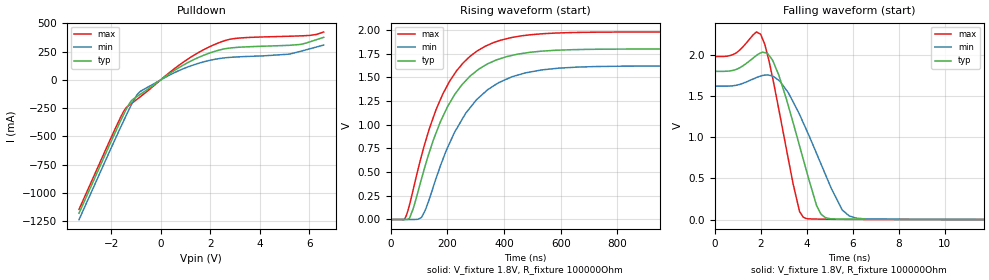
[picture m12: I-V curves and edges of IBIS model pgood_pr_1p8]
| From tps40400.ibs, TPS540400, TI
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|   pgood_pr_1p8 Model
[Model]   pgood_pr_1p8
Model_type   Open_drain
Polarity   Non-Inverting
Vmeas = 0.9
Vref = 1.8
Cref = 1pF
Rref = 100000
|   typ   min   max
C_comp   1.431pF   1.292pF   1.756pF
[Voltage Range]   3.3   3.2   3.4
[Temperature Range]   25   125   -40
[Pullup Reference]   3.3   3.2   3.4
[Pulldown Reference]   -0   -0   -0
[Power Clamp Reference]   3.3   3.2   3.4
[GND Clamp Reference]   -0   -0   -0
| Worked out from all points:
|   slope of the pulldown table from 0 to 0.495 V, typ, clamps not added: 6.57 ohm
|   falling waveform, V_fixture 1.8V, R_fixture 100000Ohm: 20-80 % time 1.09ns typ, 1.51ns min, 824ps max; typ from 1.8 V to 0 V
|   rising waveform, V_fixture 1.8V, R_fixture 100000Ohm: 20-80 % time 154ns typ, 167ns min, 151ns max; typ from 0 V to 1.8 V
[Pulldown]
|   Voltage   I(typ)   I(min)   I(max)
-3.3V     -1.181A    -1.238A    -1.147A
-1.518V   -316.1mA   -372.4mA   -288mA
-1.379V   -254.8mA   -308mA     -243.1mA
-1.171V   -181.7mA   -215.2mA   -207.3mA
-825mV    -127.7mA   -102mA     -149.2mA
976.8mV   138.9mA    104.5mA    166.5mA
1.769V    221mA      161.9mA    271.1mA
2.501V    271.5mA    193.4mA    341.5mA
3.194V    289.9mA    204.9mA    371.3mA
5.194V    306.5mA    228.3mA    386.9mA
5.848V    324.5mA    264.9mA    392.1mA
6.59V     377.4mA    308.9mA    424.9mA
[Ramp]
R_load = 100000
|   typ   min   max
dV/dt_r   1.07992/1.54451e-07   0.971899/1.66513e-07   1.18792/1.50633e-07
dV/dt_f   1.07992/1.08763e-09   0.971899/1.50929e-09   1.18792/8.24371e-10
[Falling Waveform]
V_fixture = 1.8V
V_fixture_min = 1.62V
V_fixture_max = 1.98V
R_fixture = 100000Ohm
C_fixture = 0F
|   Time   V(typ)   V(min)   V(max)
0s        1.8V       1.62V      1.98V
1.999ns   2.023V     1.742V     2.25V
2.359ns   1.995V     1.754V     1.932V
2.791ns   1.752V     1.69V      1.335V
3.409ns   1.177V     1.429V     435mV
3.845ns   738.6mV    1.18V      32.11mV
4.62ns    66.86mV    676.3mV    6.94mV
5.54ns    7.701mV    118.9mV    4.249mV
6.91ns    4.713mV    9.257mV    2.715mV
3us       138.7uV    167.9uV    129.2uV
[Rising Waveform]
V_fixture = 1.8V
V_fixture_min = 1.62V
V_fixture_max = 1.98V
R_fixture = 100000Ohm
C_fixture = 0F
|   Time   V(typ)   V(min)   V(max)
0s        138.7uV    167.9uV    129.2uV
51.66ns   -612.4uV   -264.9uV   18.31mV
66.38ns   14.12mV    -188.3uV   154.1mV
109.1ns   433.7mV    22.58mV    677mV
160.4ns   916mV      437mV      1.163V
208.2ns   1.23V      807.7mV    1.461V
302.7ns   1.568V     1.264V     1.775V
425.2ns   1.731V     1.504V     1.921V
732.1ns   1.797V     1.615V     1.978V
3us       1.8V       1.62V      1.98V
